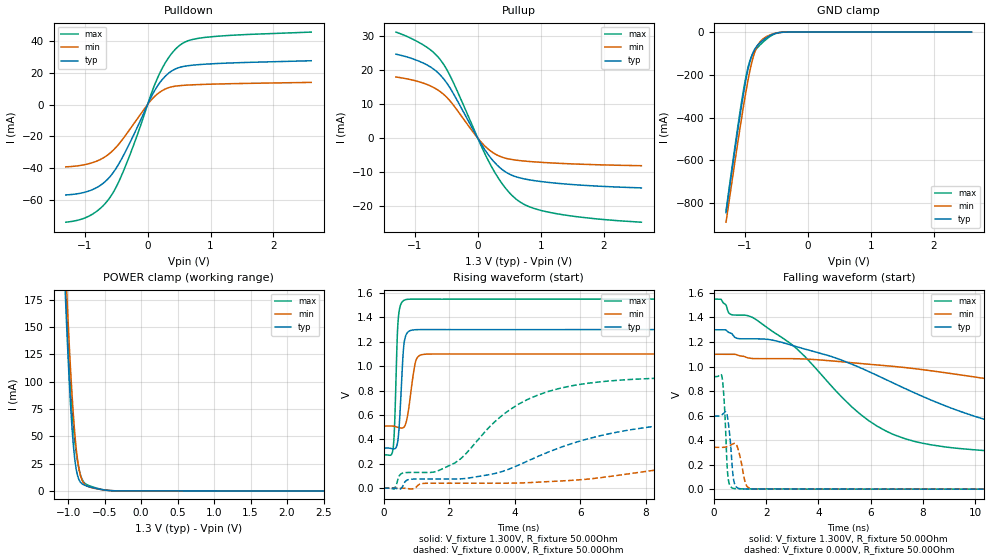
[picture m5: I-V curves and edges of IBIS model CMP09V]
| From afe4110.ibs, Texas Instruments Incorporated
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|   CMP09V  model
[Model]   CMP09V
Model_type   I/O
Vinl =  0.39V |0.275V for 1.1V
Vinh =  0.91V |0.825V for 1.1V
Vmeas = 1.500V
Cref = 25pF |25pF for VDD=1.55V; 15pF for VDD=1.1V
|   typ   min   max
|   (weak)   (typ)   (fast)
C_comp   0.7792pF   0.7756pF   0.7828pF
[Model Spec]
Vinl   0.39V   0.275V   0.465V
Vinh   0.91V   0.825V   1.085V
[Voltage Range]   1.300V   1.100V   1.550V
[Temperature Range]   27.0   85.0   0.0
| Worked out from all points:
|   slope of the pulldown table from 0 to 0.195 V, typ, clamps not added: 14.2 ohm
|   slope of the pullup table from 0 to 0.195 V, typ, clamps not added: 34.9 ohm
|   GND clamp passes 1 mA (typ) near -0.42 V on its own axis
|   POWER clamp passes 1 mA (typ) near -0.52 V on its own axis
|   falling waveform, V_fixture 1.300V, R_fixture 50.00Ohm: 20-80 % time 7.05ns typ, 13.5ns min, 3.95ns max; typ from 1.3 V to 0.329 V
|   rising waveform, V_fixture 1.300V, R_fixture 50.00Ohm: 20-80 % time 118ps typ, 182ps min, 89.2ps max; typ from 0.329 V to 1.3 V
|   rising waveform, V_fixture 0.000V, R_fixture 50.00Ohm: 20-80 % time 4.12ns typ, 7.42ns min, 2.46ns max; typ from 0 V to 0.596 V
|   falling waveform, V_fixture 0.000V, R_fixture 50.00Ohm: 20-80 % time 141ps typ, 191ps min, 119ps max; typ from 0.596 V to 0 V
[Pulldown]
|   Voltage   I(typ)   I(min)   I(max)
-1.3V     -56.75mA   -39.13mA   -73.85mA
-888.4mV  -53.62mA   -36.64mA   -69.09mA
-712.1mV  -49.6mA    -33.68mA   -63.7mA
-574.9mV  -44.18mA   -29.74mA   -56.96mA
-457.3mV  -37.25mA   -24.83mA   -48.37mA
-320.1mV  -27.06mA   -17.66mA   -35.55mA
150.3mV   11.21mA    6.413mA    15.97mA
326.6mV   19.39mA    10.45mA    29mA
522.6mV   23.44mA    11.87mA    37.5mA
718.6mV   24.69mA    12.35mA    40.85mA
1.032V    25.56mA    12.78mA    42.57mA
2.6V      27.46mA    13.88mA    45.44mA
[GND Clamp]
|   Voltage   I(typ)   I(min)   I(max)
-1.3V     -845.2mA   -890mA     -836.4mA
-1.182V   -599.5mA   -653.6mA   -585.5mA
-1.084V   -402.5mA   -462mA     -385.6mA
-1.026V   -292.7mA   -352.4mA   -276.1mA
-966.8mV  -196.6mA   -250.9mA   -184.9mA
-908mV    -125.2mA   -163.6mA   -124.2mA
-849.2mV  -82.6mA    -98.89mA   -90.41mA
-790.5mV  -58.8mA    -58.92mA   -69.47mA
-712.1mV  -38.29mA   -31.66mA   -46.82mA
-535.7mV  -7.965mA   -6.689mA   -9.902mA
-378.9mV  -410.6uA   -401.1uA   -524.8uA
2.6V      0A         0A         0A
[Pullup]
|   Voltage   I(typ)   I(min)   I(max)
-1.3V     24.77mA    18.03mA    31.28mA
-829.6mV  21.82mA    15.98mA    27.07mA
-672.9mV  19.94mA    14.63mA    24.76mA
-555.3mV  17.78mA    13.11mA    22.12mA
-378.9mV  12.86mA    9.547mA    16.05mA
0V        193.8nA    138.7nA    226.6nA
169.8mV   -4.968mA   -3.301mA   -6.724mA
405mV     -9.522mA   -5.753mA   -13.91mA
620.6mV   -11.49mA   -6.541mA   -18.18mA
855.8mV   -12.44mA   -6.966mA   -20.53mA
1.209V    -13.25mA   -7.378mA   -22.18mA
2.6V      -14.71mA   -8.161mA   -24.83mA
[POWER Clamp]
|   Voltage   I(typ)   I(min)   I(max)
-1.3V     673.1mA    684.4mA    699mA
-1.045V   190.9mA    222.2mA    206.2mA
-1.026V   159.5mA    192.1mA    174.3mA
-1.006V   130mA      163.4mA    144.4mA
-966.8mV  78.74mA    111.5mA    93.68mA
-927.6mV  41.24mA    68.99mA    57.66mA
-908mV    28.45mA    52.06mA    44.8mA
-868.8mV  13.5mA     27.37mA    26.16mA
-810.1mV  6.517mA    9.885mA    10.71mA
-712.1mV  3.812mA    3.572mA    4.78mA
-398.5mV  154.7uA    187.5uA    190.9uA
2.6V      -36.78uA   -23.84uA   -58.74uA
[Ramp]
R_load = 50.00Ohm
|   typ   min   max
dV/dt_r   357.465mV/4.117ns   204.669mV/7.415ns   550.571mV/2.455ns
dV/dt_f   582.793mV/7.032ns   354.279mV/13.447ns  766.389mV/3.948ns
[Falling Waveform]
V_fixture = 1.300V
V_fixture_min = 1.100V
V_fixture_max = 1.550V
R_fixture = 50.00Ohm
|   Time   V(typ)   V(min)   V(max)
0s        1.3V       1.1V       1.55V
2.9ns     1.179V     1.064V     1.193V
5.27ns    1.02V      1.031V     672.6mV
6.55ns    897mV      1.007V     477.7mV
8.29ns    728.2mV    965.9mV    362.3mV
11.36ns   512.1mV    870.2mV    303.6mV
15ns      400mV      758.7mV    283.1mV
20.72ns   348.8mV    634.4mV    274.3mV
33.77ns   329.2mV    530.3mV    272.5mV
125ns     328.7mV    509.5mV    272.7mV
[Rising Waveform]
V_fixture = 1.300V
V_fixture_min = 1.100V
V_fixture_max = 1.550V
R_fixture = 50.00Ohm
|   Time   V(typ)   V(min)   V(max)
0s        328.7mV    509.5mV    272.7mV
290ps     322.9mV    508.9mV    328.6mV
340ps     323.7mV    506.1mV    561.7mV
420ps     368.3mV    500mV      1.271V
480ps     532.5mV    495.8mV    1.463V
620ps     1.179V     500.8mV    1.54V
790ps     1.289V     701.7mV    1.549V
1ns       1.299V     1.057V     1.55V
1.41ns    1.3V       1.099V     1.549V
125ns     1.3V       1.1V       1.55V
[Rising Waveform]
V_fixture = 0.000V
V_fixture_min = 0.000V
V_fixture_max = 0.000V
R_fixture = 50.00Ohm
|   Time   V(typ)   V(min)   V(max)
0s        388.9uV    395.4uV    454.7uV
320ps     209.1uV    548.4uV    -7.868mV
570ps     10.1mV     265uV      122.6mV
2.17ns    75.18mV    41.28mV    206.6mV
3.58ns    133.5mV    41.16mV    588.4mV
4.7ns     259.3mV    49.3mV     762.5mV
8.91ns    526.1mV    169.5mV    905.8mV
14.84ns   588.6mV    292.3mV    918.2mV
23.32ns   596.4mV    334.6mV    918.1mV
125ns     596.2mV    341.5mV    918.1mV
[Falling Waveform]
V_fixture = 0.000V
V_fixture_min = 0.000V
V_fixture_max = 0.000V
R_fixture = 50.00Ohm
|   Time   V(typ)   V(min)   V(max)
0s        596.2mV    341.5mV    918.1mV
320ps     607.5mV    341.3mV    908.4mV
410ps     625.6mV    342.3mV    672.6mV
490ps     620.1mV    346.2mV    277mV
590ps     480.7mV    354.4mV    46.21mV
750ps     88.89mV    371.3mV    6.435mV
900ps     11.95mV    345.9mV    3.462mV
1.24ns    1.683mV    33.46mV    2.701mV
1.65ns    1.776mV    1.451mV    2.614mV
125ns     388.9uV    395.4uV    454.7uV
